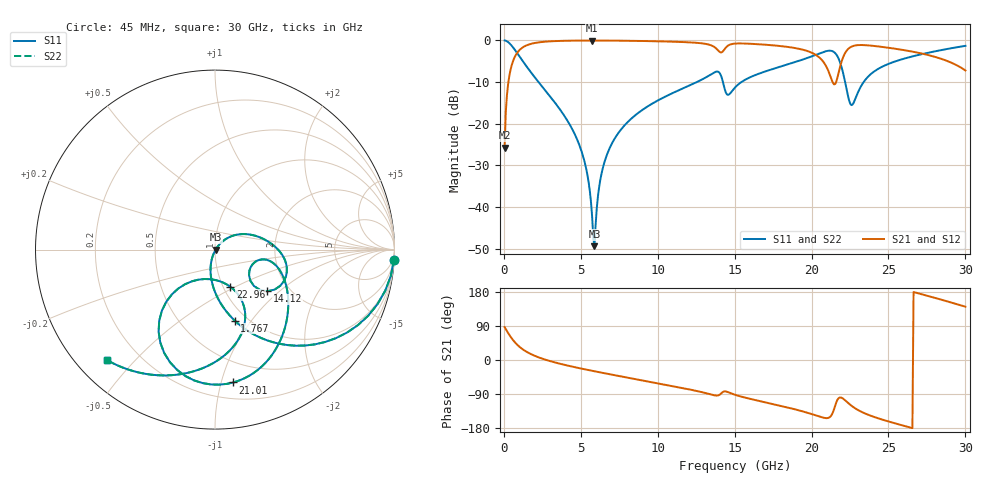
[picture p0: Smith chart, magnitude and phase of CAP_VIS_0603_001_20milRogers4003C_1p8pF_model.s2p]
! S-parameter model data by Modelithics Inc.  support@modelithics.com  813-866-6335  Tampa FL USA
! S-Parameter data specifications:
! Substrate: 20-mil Rogers 4003C, substrate thickness, H=0.508mm, Dielectric constant, Er=3.75
! PCB Mounting Pad Footprint: Pad width, PadW=0.90mm , Pad length, PadL=1.00mm , Pad gap, PadG (edge-to-edge)=1.00mm , Reference planes=3.0mm apart
! Created Wed Nov 18 13:19:09 2015
# hz S ma R 50
! 2 Port Network Data from SP1.SP block
! freq  magS11  angS11  magS21  angS21  magS12  angS12  magS22  angS22
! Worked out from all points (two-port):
!   401 points, 45 MHz to 30 GHz, reference 50 ohm
!   highest |S21| = -0.03 dB at 5.736 GHz (marker M1); lowest = -25.8 dB at 45 MHz (marker M2)
!   |S21| within 3 dB of the highest: 854.1 MHz to 20.05 GHz (19.2 GHz wide, 184 % of centre); 22.18 GHz to 27.01 GHz (4.828 GHz wide, 19.6 % of centre)
!   lowest |S11| = -49.4 dB at 5.886 GHz (marker M3), VSWR 1.01, Z = 50.3 - j0.0563 ohm
!   |S11| at or under -10 dB: 2.249 GHz to 12.55 GHz (10.3 GHz wide, 139 % of centre); 14.24 GHz to 15.44 GHz (1.205 GHz wide, 8.12 % of centre); 22.18 GHz to 23.39 GHz (1.205 GHz wide, 5.29 % of centre)
!   |S22| runs from -49.4 to 0.0 dB; largest |S21 - S12| = 0
!   S11 on the Smith chart (normalised r, x): 45 MHz: 1, -36; 1.767 GHz: 0.88, -0.83; 14.12 GHz: 1.55, -0.84; 21.01 GHz: 0.33, -1.09; 22.96 GHz: 1.08, -0.47; 30 GHz: 0.09, -0.42
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4.5e7  0.9987 -3.2  0.05145 86.8  0.05145 86.8  0.9987 -3.2
2.696625e8  0.9553 -18.6  0.2955 71.4  0.2955 71.4  0.9553 -18.6
5.692125e8  0.8353 -36.2  0.5492 53.8  0.5492 53.8  0.8353 -36.2
1.767412e9  0.411 -74.4  0.9099 15.3  0.9099 15.3  0.411 -74.4
5.062462e9  0.04561 -109.3  0.9956 -22.9  0.9956 -22.9  0.04561 -109.3
5.4369e9  0.02371 -108.7  0.9962 -26.1  0.9962 -26.1  0.02371 -108.7
5.73645e9  0.007551 -94.1  0.9964 -28.5  0.9964 -28.5  0.007551 -94.1
5.886225e9  0.003376 -9.5  0.9963 -29.8  0.9963 -29.8  0.003376 -9.5
6.33555e9  0.0246 48.9  0.9958 -33.3  0.9958 -33.3  0.0246 48.9
7.009538e9  0.05726 47.8  0.9942 -38.6  0.9942 -38.6  0.05726 47.8
1.007992e10  0.1932 26.5  0.9753 -62.0  0.9753 -62.0  0.1932 26.5
1.285076e10  0.3372 2.4  0.9232 -84.7  0.9232 -84.7  0.3372 2.4
1.412385e10  0.3732 -38.4  0.7157 -88.1  0.7157 -88.1  0.3732 -38.4
1.50225e10  0.2715 -11.6  0.9157 -91.7  0.9157 -91.7  0.2715 -11.6
2.003996e10  0.6462 -58.0  0.7073 -143.1  0.7073 -143.1  0.6462 -58.0
2.10135e10  0.7473 -82.2  0.4627 -153.4  0.4627 -153.4  0.7473 -82.2
2.146282e10  0.7236 -103.1  0.2965 -129.6  0.2965 -129.6  0.7236 -103.1
2.183726e10  0.5546 -124.5  0.4684 -98.9  0.4684 -98.9  0.5546 -124.5
2.251125e10  0.174 -109.6  0.8253 -118.0  0.8253 -118.0  0.174 -109.6
2.296058e10  0.2245 -67.5  0.876 -130.7  0.876 -130.7  0.2245 -67.5
2.505742e10  0.5275 -76.6  0.8131 -162.9  0.8131 -162.9  0.5275 -76.6
3e10  0.8602 -134.2  0.4356 140.7  0.4356 140.7  0.8602 -134.2
